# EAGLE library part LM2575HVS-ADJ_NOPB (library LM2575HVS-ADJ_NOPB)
IC,regulator,voltage,switching,step-down,adjustable,TO263-5,LM2575HVS-ADJ/NOPB Source: Datasheet
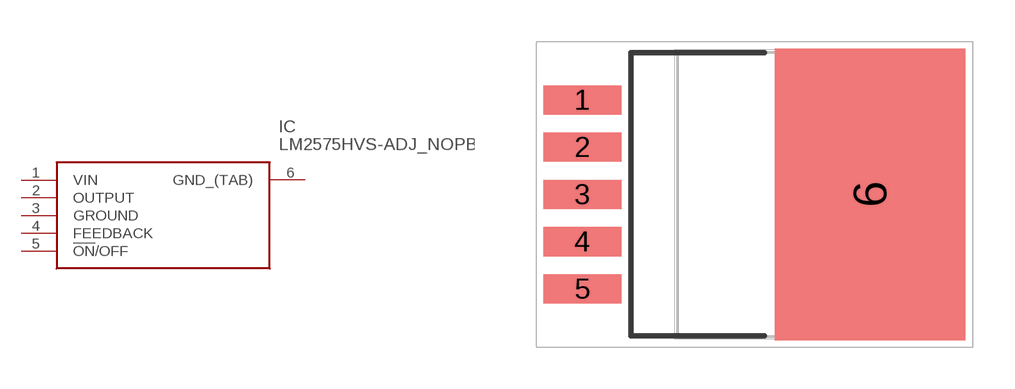
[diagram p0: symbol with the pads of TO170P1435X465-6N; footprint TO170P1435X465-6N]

Designator prefix IC

## LM2575HVS-ADJ_NOPB (Description: IC,regulator,voltage,switching,step-down,adjustable,TO263-5,LM2575HVS-ADJ/NOPB; Height: 4.65mm; Manufacturer_Name: Texas Instruments; Manufacturer_Part_Number: LM2575HVS-ADJ/NOPB; Mouser_Part_Number: 926-LM2575HVSADJNOPB; Mouser_Price-Stock: https://www.mouser.co.uk/ProductDetail/Texas-Instruments/LM2575HVS-ADJ-NOPB?qs=X1J7HmVL2ZH4Vy9jY3DJlQ%3D%3D)  [TO170P1435X465-6N]
1  VIN  in
2  OUTPUT  out
3  GROUND
4  FEEDBACK
5  !ON!/OFF
6  GND_(TAB)  pwr

## Footprint TO170P1435X465-6N (pad centres in mm)
KTT0005B
smd 2.8 x 1.05: 1 -6.2,3.4; 2 -6.2,1.7; 3 -6.2,0; 4 -6.2,-1.7; 5 -6.2,-3.4
smd 6.85 x 10.5: 6 4.15,0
